(* Logix 5000 AddOnInstructionDefinition export T2HC; software revision 32.02 *)

TYPE Exlar_Control :   // Tritex II Control
STRUCT
   EnableOutputs : INT;   // EnableOutputs
   InputEventsMode : INT;   // 4316
   InputEventsModeLevel : INT;   // 4318
   InputEventsMotion : INT;   // 4317
   HostCommandControlMode : INT;   // 4303
   HostPosition_low : INT;   // 4304
   HostPosition_high : INT;
   HostVelocity_low : INT;   // 4306
   HostVelocity_high : INT;
   HostAcceleration_low : INT;   // 4308
   HostAcceleration_high : INT;
   HostCurrent : INT;   // 4310
   InputEventsMoveEdge : INT;   // 4319
   JogSlowVelocity_low : INT;   // 6022
   JogSlowVelocity_high : INT;
   JogAcceleration_low : INT;   // 6026
   JogAcceleration_high : INT;
   MoveOption : INT;   // 6100
   MoveCurrentLimit : INT;   // 6101
   MoveAcceleration_low : INT;   // 6102
   MoveAcceleration_high : INT;
   MoveDeceleration_low : INT;   // 6500
   MoveDeceleration_high : INT;
   MovePrimaryOption : INT;   // 6106
   spare : INT;   // spare
   MovePrimaryPosition_low : INT;   // 6108
   MovePrimaryPosition_high : INT;
   MovePrimaryVelocity_low : INT;   // 6110
   MovePrimaryVelocity_high : INT;
   MoveSecondaryOption : INT;   // 6112
   spare2 : INT;   // spare
   MoveSecondaryPosition_low : INT;   // 6114
   MoveSecondaryPosition_high : INT;
   MoveSecondaryVelocity_low : INT;   // 6116
   MoveSecondaryVelocity_high : INT;
END_STRUCT
END_TYPE

TYPE Exlar_Drive :   // Tritex II Data
STRUCT
   Control : Exlar_Control;   // Control bits to send to the drive
   Status : Exlar_Status;   // Status bits received from the drive
END_STRUCT
END_TYPE

TYPE Exlar_Status :   // Tritex II Status
STRUCT
   EIP_Comm : INT;   // EIP module communication
   OutputEventsStatus : INT;   // 104
   OutputEventsMoveInPosition : INT;   // 108
   OutputEventsMotion : INT;   // 105
   OutputsEventsMotionActive : INT;   // 107
   PositionFeedback_low : INT;   // 378
   PositionFeedback_high : INT;
   SoftFaults : INT;   // 7
   HardFaults : INT;   // 6
   VelocityDisplay_low : INT;   // 356
   VelocityDisplay_high : INT;
   CurrentDisplay : INT;   // 567
   CurrentContinuous : INT;   // 565
   CurrentLimit : INT;   // 5108
   VoltageHallBattery : INT;   // 8
   VoltageBus : INT;   // 571
   TemperatureBoard : INT;   // 11
   TemperatureActuator : INT;   // 15
END_STRUCT
END_TYPE

ADD_ON_INSTRUCTION T2HC   (* revision 1.1, vendor Exlar Corporation *)
// Help:
// Use the Tritex 2 HC(T2HC) instruction to control drive Host Control Option
// Configured for Exlar EIP AOI. 07/01/2014
// ----------------------------------------------------------------------------------------------------------------------------
// Parameters Bit Definition
// ----------------------------------------------------------------------------------------------------------------------------
// CommandMode:   (Input) Control Host Mode
// ------------------------------------------------------------------
//    0 = Disable Host Control
//    5 = Position
//    6 = Velocity
//    7 = Current
VAR_IN_OUT
   Drive : Exlar_Drive; {required}   // Drive
   Units : REAL[5]; {required}   // Units
END_VAR
VAR_INPUT
   CommandMode : INT; {visible}   // Host Control
   Position : REAL; {visible}   // Position
   Velocity : REAL; {visible}   // Velocity
   Acceleration : INT; {visible}   // Acceleration
   Current : REAL; {visible}   // Current
END_VAR
VAR_OUTPUT
   DF : BOOL; {access Read Only, visible}   // A Drive Fault is active
   ER : BOOL; {access Read Only, visible}   // A Instruction error is Active
END_VAR
VAR
   tempDINT : DINT; {access None}   // Temporary Register used in calculating units
END_VAR

ROUTINE Logic   (* structured text *)
   (***********************************************)
   (*   Exlar Tritex 2 Host Control               *)
   (*                                             *)
   (***********************************************)
   
   
   (* Precondition  *)
   	ER	:= 0;
   
   (* Check valid Host Control *)
   	(* CommandMode
   		 0 = Disabled
            5 = Position
            6 = Velocity
            7 = Current
   	*)
   	if CommandMode = 0 OR CommandMode = 5
   		OR CommandMode = 6 OR CommandMode = 7 then
   
   		(* ID:4303, Control.Host.CommandMode:  Outputs[4]] *)
   		Drive.Control.HostCommandControlMode := CommandMode;
   	else
   		ER	:= 1;
   		Drive.Control.HostCommandControlMode := 0;
   	end_if;
   
   
   (********** Outputs **********)
   (* Drive Faults Active *)
   	(* 104.03 Fault *)
   	if Drive.Status.OutputEventsStatus.3 then
    		DF := 1;
   	Else
   		DF := 0;
   	End_If;
   
   
   (* Error Test *)
   	(* User Units Instruction error active ? *)
   	IF Units[0] = 0 THEN
   		ER	:= 1;
   	end_if;
   
   (* Update Units *)
   	if NOT ER  then
   
   		(* Position *)
   		(* ID:4304, Control.Host.Postion:  ModuleOutputs[6],ModuleOutputs[5] *)
   		tempDINT := Position / Units[1];
   		cps(tempDINT, Drive.Control.HostPosition_low,2);
   
   		(* Velocity *)
   		(* ID:4306, Control.Host.Velocity:  ModuleOutputs[8],ModuleOutputs[7] *)
   		tempDINT := Velocity / Units[2];
   		cps(tempDINT, Drive.Control.HostVelocity_low,2);
   
   		(* Acceleration *)
   		(* ID:4308, Control.Host.Acceleration:  ModuleOutputs[10],ModuleOutputs[9] *)
   		tempDINT := Acceleration / Units[3];
   		cps(tempDINT, Drive.Control.HostAcceleration_low,2);
   
   		(* Current Scale   *)
   		(*       0: AMPs   *)
   		(*       1: %      *)
   		(* ID:4310, Control.Host.Current:  ModuleOutputs[11] *)
   		if Units[4] = 0	then
   			Drive.Control.HostCurrent := Current / 0.0078125 ;
   		else
   			(* Use for % ,ID:5108, Config.CurrentLimit:   ModuleInputs[13],  *)
   			Drive.Control.HostCurrent := Drive.Status.CurrentLimit * (Current /100);
   		end_if;
   
   	end_if;
   
   
   
END_ROUTINE
END_ADD_ON_INSTRUCTION
